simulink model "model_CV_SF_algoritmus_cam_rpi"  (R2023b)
settings: Solver=FixedStepAuto  StartTime=0.0  StopTime=inf  RelTol=1e-3  EnableMultiTasking=on
undefined symbols (not defined in the file): adaptor, C, Camera, genericvideo, HD, HP, imaq, MATLAB, Newmine, none, ProgramData, R2023b, SupportPackages, supportpackages, toolbox, videoinput, win64, winvideo
libraries: visionsinks x2, lib_control_system_SF x1, imaqlib x1, deeplib x1, visiontextngfix x1, dspstat3 x1, raspberrypiBasiclib x1

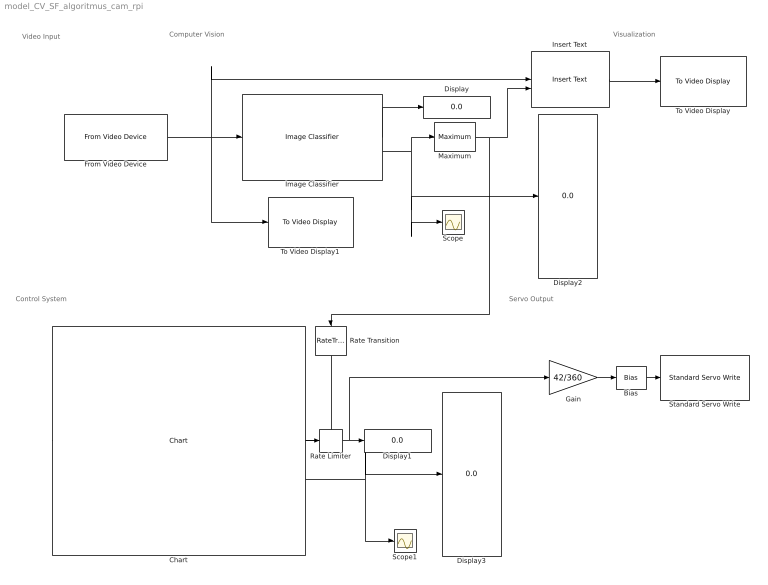
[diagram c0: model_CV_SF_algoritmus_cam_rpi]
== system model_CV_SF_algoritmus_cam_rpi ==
  note: Video Input
  note: Servo Output
  note: Control System
  note: Computer Vision
  note: Visualization
  Bias : Bias  Bias=2
  Chart : lib_control_system_SF/Chart  SystemSampleTime=-1  VariantActivationTime=update diagram  AllowFlexibleInterface=on  Latency=0  AutoFrameSizeCalculation=off
  Display{,1..3} (4 alike) : Display
  From Video Device : imaqlib/From Video Device  DeviceMenu=winvideo 1 (HP HD Camera)  Device=winvideo 2 (Newmine Camera)  ObjConstructor=videoinput('winvideo', 2)  VideoFormatMenu=MJPG_320x240  VideoFormat=MJPG_320x240  VideoSource=input1  ROIPosition=[0 0 240 320]  EnableHWTrigger=off  TriggerConfiguration=none/none  SampleTime=1/10  OutputPortsMode=One multidimensional signal  DataType=uint8  CanDoHWTrigger=no  ReturnedColorSpace=rgb  BlockHandle=214.0046  ROIWidth=320  ROIHeight=240  ROIColumn=0  ROIRow=0  EngXMLPath=C:\Program Files\MATLAB\R2023b\toolbox\imaq\imaq\private  DevXMLPath=C:\ProgramData\MATLAB\SupportPackages\R2023b\toolbox\imaq\supportpackages\genericvideo\adaptor\win64  EngLibPath=C:\Program Files\MATLAB\R2023b\toolbox\imaq\imaqblks\imaqmex\win64  ColorSpace=rgb  BayerSensorAlignment=grbg  ImaqMode=off
  Gain : Gain  Gain=42/360
  Image Classifier : deeplib/Image Classifier  Network=Network from MAT-file  NetworkFunction=squeezenet  NetworkFilePath=trainedNetwork.mat  MiniBatchSize=8  ResizeInput=on  Classification=on  Predictions=on  ForceInterpretedSim=off  PredictMode=All probabilities and labels  K=5
  Insert Text : visiontextngfix/Insert Text  inputType=Obsolete  theText={'Hmozdinka','Hrebik','Matice','Matice kridlova','Podlozka','Prazdne','Sroub','Vrut'}  getTextLocFrom=Specify via dialog  textLoc=[1 1]  getTextColorFrom=Specify via dialog  textColor=[0 0 0]  getTextIntensityFrom=Specify via dialog  textIntensity=0  getTextOpacityFrom=Specify via dialog  textOpacity=1.0  dummyVar2=0  dummyVar3=0  dummyVar4=0  imagePorts=One multidimensional signal  isInputTransposed=off  fontFace=LucidaSansRegular  dummyVar1=0  blockFontSize=32  antiAliased=on
  Maximum : dspstat3/Maximum  operation=maximum  fcn=Index  indexBase=One  operateOver=Each row  Dimension=1  InputProcessing=Columns as channels (frame based)  reset=None  roiEnable=off  roiType=Rectangles  roiPortion=Entire ROI  roiOutput=Individual statistics for each ROI  roiFlag=off  roundingMode=Floor  overflowMode=off  accumDataTypeStr=Inherit: Same as product output  accumLastDataTypeStr=Inherit: Same as product output
  Rate Limiter : RateLimiter  RisingSlewLimit=15  FallingSlewLimit=-15  SampleTimeMode=inherited
  Rate Transition : RateTransition  OutPortSampleTime=0.1
  Scope : Scope
  Scope1 : Scope
  Standard Servo Write : raspberrypiBasiclib/Standard Servo Write  board=Pi 2 Model B  Pin_=18  MinPulseDuration=1000e-6  MaxPulseDuration=2000e-6  blockPlatform=Raspberry Pi
  To Video Display : visionsinks/To Video Display  windowSizeMode=Normal  openAtMdlStart=on  fullScreen=off  videoWindowX=1368  videoWindowY=406  saveWindowSize=off  videoWindowWidth=227  videoWindowHeight=227  inputColorFormat=RGB  inputType=Obsolete  imagePorts=One multidimensional signal  OutputDevice=On-screen video monitor  dataOrg=Column-major  isWindowOpen=off
  To Video Display1 : visionsinks/To Video Display  windowSizeMode=Normal  openAtMdlStart=on  fullScreen=off  videoWindowX=1136  videoWindowY=407  saveWindowSize=off  videoWindowWidth=227  videoWindowHeight=227  inputColorFormat=RGB  inputType=Obsolete  imagePorts=One multidimensional signal  OutputDevice=On-screen video monitor  dataOrg=Column-major  isWindowOpen=off
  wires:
  From Video Device/1 -> Image Classifier/1, Insert Text/1, To Video Display1/1
  Image Classifier/1 -> Display/1
  Image Classifier/2 -> Maximum/1, Scope/1, Display2/1
  Insert Text/1 -> To Video Display/1
  Maximum/1 -> Insert Text/2, Rate Transition/1
  Chart/1 -> Rate Limiter/1
  Chart/2 -> Display3/1, Scope1/1
  Gain/1 -> Bias/1
  Bias/1 -> Standard Servo Write/1
  Rate Limiter/1 -> Gain/1, Display1/1
  Rate Transition/1 -> Chart/1
